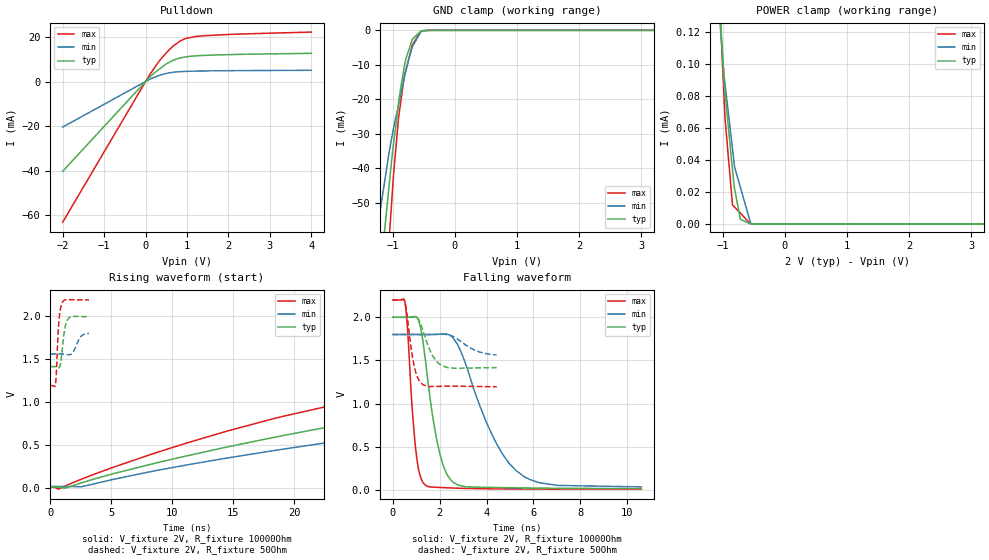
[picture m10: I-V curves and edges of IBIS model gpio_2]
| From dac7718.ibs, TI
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|   gpio_2 Model
[Model]   gpio_2
Model_type   I/O_open_drain
Polarity   Non-Inverting
Enable   Active-Low
Vinl = 0.3
Vinh = 1.5
Vmeas = 1.0
Vref = 2.0
Cref = 15pF
Rref = 10000
|   typ   min   max
|   (nom PVT)   (Fast PVT)   (slow PVT)
|C_comp from Frequency method(F=50MHz)
|Average
|C_comp   4.052e-12   3.350e-12   4.556e-12
|OFF state: BUFFER IN HIGH IMPEDANCE
|C_comp   3.811e-12   3.136e-12   4.352e-12
|ON state : BUFFER OUTPUT TURNED LOW
C_comp   4.294e-12   3.563e-12   4.761e-12
|C_comp from LC Tank Method (L=1nH)
|Resonant Frequency(Hz)   2.906e9   3.12e9   2.82e9
|C_comp   2.894e-12   2.605e-12   3.188e-12
| Where nom  PVT is Nominal Process,  2V,  33C
|   Fast PVT is Strong Process,   2.2V,  -40C
|   Slow PVT is Weak Process,   1.8V,  113C
[Voltage Range]   2   1.8   2.2
[Temperature Range]   33   113   -40
[Pullup Reference]   2   1.8   2.2
[Pulldown Reference]   0   0   0
[Power Clamp Reference]   2   1.8   2.2
[GND Clamp Reference]   0   0   0
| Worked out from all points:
|   slope of the pulldown table from 0 to 0.3 V, typ, clamps not added: 58.7 ohm
|   GND clamp passes 1 mA (typ) near -0.59 V on its own axis
|   POWER clamp passes 1 mA (typ) near -1.80 V on its own axis
|   falling waveform, V_fixture 2V, R_fixture 10000Ohm: 20-80 % time 671ps typ, 1.63ns min, 335ps max; typ from 2 V to 0.013 V
|   rising waveform, V_fixture 2V, R_fixture 10000Ohm: 20-80 % time 89.8ns typ, 102ns min, 71.5ns max; typ from 0.01 V to 2 V
|   falling waveform, V_fixture 2V, R_fixture 50Ohm: 20-80 % time 507ps typ, 847ps min, 325ps max; typ from 2 V to 1.42 V
|   rising waveform, V_fixture 2V, R_fixture 50Ohm: 20-80 % time 303ps typ, 471ps min, 226ps max; typ from 1.41 V to 2 V
[Pulldown]
|   Voltage   I(typ)   I(min)   I(max)
-2V       -40.33mA   -20.46mA   -63.19mA
105.6mV   2.035mA    992.4uA    3.213mA
387.2mV   6.352mA    3.072mA    10.53mA
482mV     7.698mA    3.564mA    12.48mA
668.8mV   9.531mA    4.16mA     15.97mA
820.6mV   10.5mA     4.411mA    18.04mA
950.4mV   11.02mA    4.544mA    19.21mA
1.289V    11.62mA    4.703mA    20.38mA
2.077V    12.11mA    4.876mA    21.19mA
4V        12.66mA    5.044mA    22.21mA
[GND Clamp]
|   Voltage   I(typ)   I(min)   I(max)
-2V       -240.7mA   -157.7mA   -352.4mA
-1.309V   -92.41mA   -64.89mA   -134.1mA
-1.194V   -69.51mA   -51.4mA    -99.74mA
-1.12V    -56.2mA    -42.7mA    -77.59mA
-1.055V   -44.54mA   -35.11mA   -60.08mA
-1.018V   -37.93mA   -31.44mA   -50.17mA
-987.8mV  -33.06mA   -28.46mA   -42.16mA
-906.4mV  -21.19mA   -21.57mA   -25.42mA
-814mV    -10.54mA   -13.76mA   -13.43mA
-684mV    -2.575mA   -4.789mA   -4.237mA
-550mV    -257.8uA   -506.5uA   -370.5uA
4V        0A         0A         0A
[POWER Clamp]
|   Voltage   I(typ)   I(min)   I(max)
-2V       1.248mA    985.9uA    1.569mA
-1.054V   139.4uA    131.3uA    142.3uA
-979.2mV  91.16uA    93.2uA     79.61uA
-970mV    85.22uA    90.1uA     71.88uA
-963.6mV  82.65uA    87.94uA    66.51uA
-842.6mV  34uA       47.13uA    11.91uA
-818mV    24.11uA    38.84uA    10.91uA
-808.2mV  21.9uA     35.53uA    10.51uA
-716mV    2.921uA    22.98uA    6.756uA
-549mV    0A         247.4nA    0A
-536.4mV  0A         171.2nA    0A
4V        0A         0A         0A
[Ramp]
R_load = 10000
|   typ   min   max
dV/dt_r   1.19375/8.98535e-08   1.06743/1.01828e-07   1.31581/7.14717e-08
dV/dt_f   1.19405/6.70089e-10   1.06943/1.64993e-09   1.31583/3.34287e-10
[Falling Waveform]
V_fixture = 2V
V_fixture_min = 1.8V
V_fixture_max = 2.2V
R_fixture = 10000Ohm
|   Time   V(typ)   V(min)   V(max)
0s        2V         1.8V       2.2V
530ps     2V         1.8V       2.161V
970ps     2.008V     1.8V       497.2mV
1.17ns    1.899V     1.8V       162.3mV
1.41ns    1.471V     1.8V       49.94mV
2.03ns    395.6mV    1.804V     26.54mV
2.76ns    57.67mV    1.686V     18.43mV
4.05ns    28.15mV    748.3mV    11.57mV
5.24ns    22.64mV    227.3mV    9.221mV
10.6ns    12.77mV    33.46mV    7.136mV
[Rising Waveform]
V_fixture = 2V
V_fixture_min = 1.8V
V_fixture_max = 2.2V
R_fixture = 10000Ohm
|   Time   V(typ)   V(min)   V(max)
0s        9.908mV    17.6mV     6.955mV
2.55ns    59.13mV    13.11mV    101.9mV
19.18ns   612.1mV    453mV      836.6mV
34.48ns   973.6mV    748.5mV    1.197V
68.81ns   1.365V     1.176V     1.642V
96.85ns   1.569V     1.348V     1.882V
128.7ns   1.734V     1.484V     2.024V
183ns     1.875V     1.632V     2.129V
265ns     1.951V     1.724V     2.181V
700ns     1.999V     1.797V     2.2V
[Falling Waveform]
V_fixture = 2V
V_fixture_min = 1.8V
V_fixture_max = 2.2V
R_fixture = 50Ohm
|   Time   V(typ)   V(min)   V(max)
0s        2V         1.8V       2.2V
505ps     2V         1.8V       2.192V
905ps     2.004V     1.8V       1.448V
1.05ns    1.993V     1.8V       1.31V
1.255ns   1.874V     1.8V       1.226V
1.675ns   1.567V     1.8V       1.198V
2.05ns    1.448V     1.802V     1.2V
2.555ns   1.411V     1.78V      1.202V
3.645ns   1.414V     1.602V     1.197V
4.435ns   1.416V     1.563V     1.194V
[Rising Waveform]
V_fixture = 2V
V_fixture_min = 1.8V
V_fixture_max = 2.2V
R_fixture = 50Ohm
|   Time   V(typ)   V(min)   V(max)
0s        1.413V     1.561V     1.191V
420ps     1.412V     1.561V     1.201V
495ps     1.41V      1.561V     1.333V
625ps     1.402V     1.561V     1.755V
710ps     1.401V     1.561V     1.944V
960ps     1.577V     1.56V      2.154V
1.205ns   1.866V     1.557V     2.189V
1.49ns    1.975V     1.551V     2.194V
2.51ns    1.996V     1.764V     2.19V
3.17ns    1.996V     1.8V       2.19V
